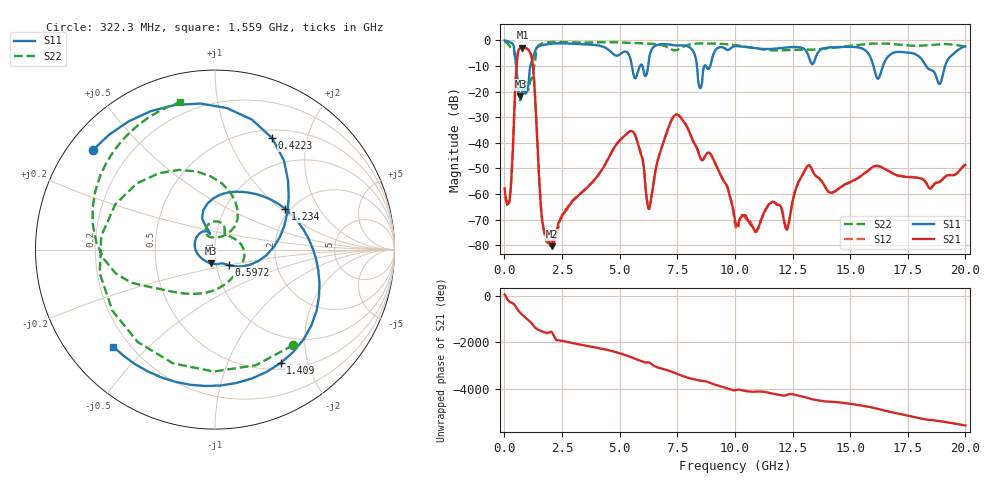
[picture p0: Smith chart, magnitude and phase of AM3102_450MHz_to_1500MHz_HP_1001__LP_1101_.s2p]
!Agilent Technologies,E8364B,MY43040894,A.07.50.67
!Agilent E8364B: A.07.50.67
!Date: Thursday, January 11, 2018 06:04:55
!Correction: S11(Full 2 Port(1,2))
!S21(Full 2 Port(1,2))
!S12(Full 2 Port(1,2))
!S22(Full 2 Port(1,2))
!S2P File: Measurements: S11, S21, S12, S22:
# Hz S  dB  R 50
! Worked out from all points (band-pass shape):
!   1601 points, 10 MHz to 20 GHz, reference 50 ohm
!   highest |S21| = -2.86 dB at 784.6 MHz (marker M1); lowest = -80.4 dB at 2.059 GHz (marker M2)
!   |S21| within 3 dB of the highest: 571.4 MHz to 1.164 GHz (592.1 MHz wide, 68.3 % of centre)
!   lowest |S11| = -21.9 dB at 697.2 MHz (marker M3), VSWR 1.18, Z = 47.1 - j7.29 ohm
!   |S11| at or under -10 dB: 513.2 MHz to 1.128 GHz (614.5 MHz wide, 74.9 % of centre); 16.01 GHz to 16.42 GHz (412 MHz wide, 2.54 % of centre); 18.29 GHz to 19.12 GHz (825.7 MHz wide, 4.41 % of centre)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
!   |S22| runs from -23.4 to -0.5 dB; largest |S21 - S12| = 0.0018
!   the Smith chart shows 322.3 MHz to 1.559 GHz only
!   S11 on the Smith chart (normalised r, x): 322.3 MHz: 0.07, +0.35; 422.3 MHz: 0.60, +1.46; 597.2 MHz: 1.14, -0.20; 1.234 GHz: 1.89, +1.08; 1.409 GHz: 0.58, -1.58; 1.559 GHz: 0.14, -0.39
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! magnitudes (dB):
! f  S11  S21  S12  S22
! 10 MHz  -0.1  -57.8  -61.2  -0.5
! 322.3 MHz  -1.1  -50.9  -51.1  -3.3
! 422.3 MHz  -3.1  -29.4  -29.5  -4.3
! 597.2 MHz  -18.8  -4.4  -4.4  -20.1
! 697.2 MHz  -21.9  -3.0  -3.0  -23.4
! 784.6 MHz  -19.3  -2.9  -2.9  -18.6
! 1.234 GHz  -6.9  -9.8  -9.8  -12.9
! 1.409 GHz  -2.7  -36.1  -36.0  -3.2
! 1.559 GHz  -2.1  -61.5  -61.9  -1.5
! 2.059 GHz  -1.3  -80.4  -79.0  -0.7
! 3.346 GHz  -1.5  -59.5  -59.4  -0.9
! 5.507 GHz  -8.9  -35.4  -35.4  -1.0
! 6.282 GHz  -7.0  -65.8  -65.6  -1.3
! 6.682 GHz  -1.7  -46.0  -46.0  -1.6
! 7.581 GHz  -2.0  -29.5  -29.5  -3.4
! 8.493 GHz  -18.7  -45.7  -45.7  -1.2
! 10.01 GHz  -2.3  -70.2  -71.8  -1.9
! 12.25 GHz  -2.8  -73.8  -73.0  -3.8
! 13.34 GHz  -9.3  -50.4  -50.4  -3.7
! 16.68 GHz  -6.1  -51.0  -51.1  -1.4
! 18.88 GHz  -17.1  -55.3  -55.4  -1.6
! 20 GHz  -2.4  -48.6  -48.8  -2.3
